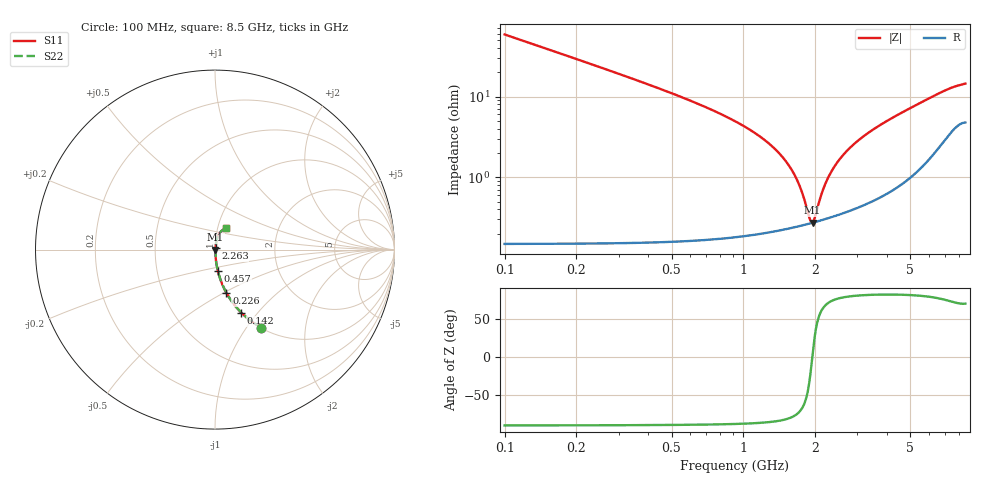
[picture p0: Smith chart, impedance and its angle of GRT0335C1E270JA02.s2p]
!Murata Part Number: GRT0335C1E270JA02
!These Parameters are Measured in Series Mode Connection
!Data Generated on Jun 19, 2026
!  o--ll--o
!Port1  Port2
!  o------o
!Operation Temp=25[degC], DC Bias Voltage=0[V]
!Freq. Start=100[MHz] Stop=9[GHz] 401[Steps]
# Hz S RI R 50
!Freq.(Hz) S11(Real) S11(Imag) S21(Real) S21(Imag) S12(Real) S12(Imag) S22(Real) S22(Imag)
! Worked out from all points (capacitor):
!   401 points, 100 MHz to 8.5 GHz, reference 50 ohm
!   read as one part in series: C = 27 pF near 142 MHz
!   lowest |Z| = 274 mohm at 1.948 GHz (marker M1)
!   series resonance near 1.942 GHz, so ESL is about 250 pH
!   S11 on the Smith chart (normalised r, x): 100 MHz: 1.00, -1.18; 142 MHz: 1.00, -0.83; 226 MHz: 1.00, -0.51; 457 MHz: 1.00, -0.24; 2.263 GHz: 1.01, +0.02; 8.5 GHz: 1.10, +0.27
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1e8  0.2574 -0.4359  0.7426 0.4359  0.7426 0.4359  0.2574 -0.4359
1.42e8  0.1466 -0.3519  0.8534 0.3519  0.8534 0.3519  0.1466 -0.3519
2.26e8  0.0633 -0.2406  0.9367 0.2406  0.9367 0.2406  0.0633 -0.2406
3.31e8  0.0304 -0.1674  0.9696 0.1674  0.9696 0.1674  0.0304 -0.1674
4.57e8  0.0161 -0.1197  0.9839 0.1197  0.9839 0.1197  0.0161 -0.1197
6.88e8  0.00722 -0.0743  0.9928 0.0743  0.9928 0.0743  0.00722 -0.0743
1.276e9  0.00275 -0.0261  0.9973 0.0261  0.9973 0.0261  0.00275 -0.0261
1.507e9  0.00251 -0.0155  0.9975 0.0155  0.9975 0.0155  0.00251 -0.0155
1.675e9  0.00252 -0.00897  0.9975 0.00897  0.9975 0.00897  0.00252 -0.00897
1.759e9  0.00256 -0.00599  0.9974 0.00599  0.9974 0.00599  0.00256 -0.00599
1.885e9  0.00266 -0.00179  0.9973 0.00179  0.9973 0.00179  0.00266 -0.00179
1.948e9  0.00273 0.000197  0.9973 -0.000197  0.9973 -0.000197  0.00273 0.000197
1.99e9  0.00278 0.00149  0.9972 -0.00149  0.9972 -0.00149  0.00278 0.00149
2.137e9  0.00298 0.00582  0.997 -0.00582  0.997 -0.00582  0.00298 0.00582
2.263e9  0.00319 0.00933  0.9968 -0.00933  0.9968 -0.00933  0.00319 0.00933
2.536e9  0.00373 0.0164  0.9963 -0.0164  0.9963 -0.0164  0.00373 0.0164
2.914e9  0.00467 0.0255  0.9953 -0.0255  0.9953 -0.0255  0.00467 0.0255
3.502e9  0.00656 0.0385  0.9934 -0.0385  0.9934 -0.0385  0.00656 0.0385
4.3e9  0.0102 0.0552  0.9898 -0.0552  0.9898 -0.0552  0.0102 0.0552
5.707e9  0.0213 0.0842  0.9787 -0.0842  0.9787 -0.0842  0.0213 0.0842
7.114e9  0.0427 0.1095  0.9573 -0.1095  0.9573 -0.1095  0.0427 0.1095
8.5e9  0.0615 0.1225  0.9385 -0.1225  0.9385 -0.1225  0.0615 0.1225
